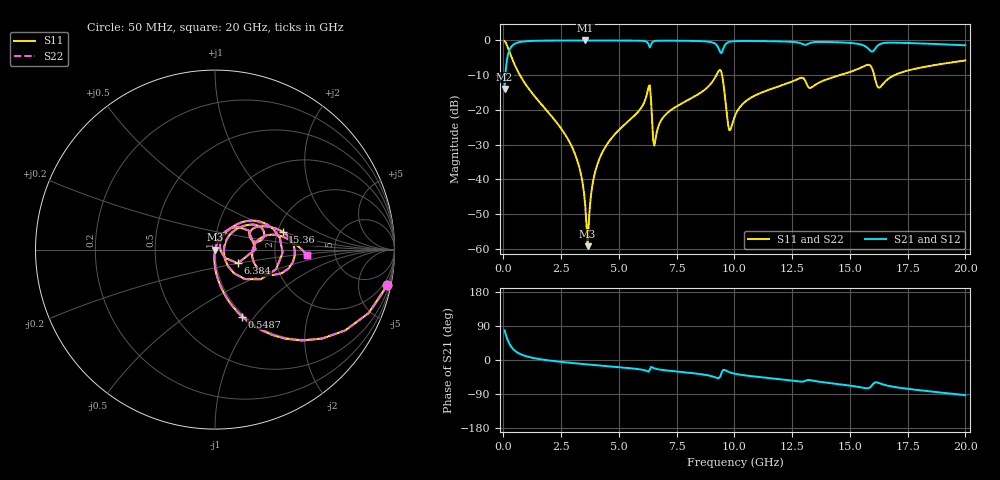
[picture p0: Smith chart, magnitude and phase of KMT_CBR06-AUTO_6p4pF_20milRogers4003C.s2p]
! Data measured by Modelithics Inc. support@modelithics.com 813-866-6335
! KEMET CBR06-AUTO 6.4pF, Pad Width= 0.851mm, Pad Length= 0.64mm, Pad Gap= 0.62mm, 20mil Rogers 4003C substrate Data, January 2022
# hz S ma R 50
! 2 Port Network Data from SP1.SP block
! freq  magS11  angS11  magS21  angS21  magS12  angS12  magS22  angS22
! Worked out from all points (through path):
!   401 points, 50 MHz to 20 GHz, reference 50 ohm
!   highest |S21| = -0.01 dB at 3.541 GHz (marker M1); lowest = -14.0 dB at 50 MHz (marker M2)
!   group delay of S21, straight-line fit = 14.4 ps
!   lowest |S11| = -59.3 dB at 3.641 GHz (marker M3), VSWR 1.00, Z = 50.1 - j0.0271 ohm
!   |S11| at or under -10 dB: 712.4 MHz to 9.218 GHz (8.505 GHz wide, 171 % of centre); 9.464 GHz to 14.57 GHz (5.107 GHz wide, 42.5 % of centre); 16.05 GHz to 16.93 GHz (880.3 MHz wide, 5.34 % of centre)
!   |S22| runs from -59.3 to -0.2 dB; largest |S21 - S12| = 0
!   S11 on the Smith chart (normalised r, x): 50 MHz: 0.98, -9.72; 548.8 MHz: 0.97, -0.87; 6.384 GHz: 1.27, -0.20; 15.36 GHz: 2.13, +0.50; 20 GHz: 3.09, -0.27
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5e7  0.98 -11.6  0.1989 78.4  0.1989 78.4  0.98 -11.6
2.495e8  0.7009 -46.3  0.7128 43.7  0.7128 43.7  0.7009 -46.3
5.4875e8  0.4021 -68.0  0.915 21.9  0.915 21.9  0.4021 -68.0
2.74325e9  0.04027 -95.1  0.9981 -6.5  0.9981 -6.5  0.04027 -95.1
3.391625e9  0.01028 -94.5  0.9988 -10.3  0.9988 -10.3  0.01028 -94.5
3.54125e9  0.004197 -86.4  0.9988 -11.1  0.9988 -11.1  0.004197 -86.4
3.641e9  0.001085 -14.4  0.9988 -11.7  0.9988 -11.7  0.001085 -14.4
3.94025e9  0.01162 71.1  0.9987 -13.3  0.9987 -13.3  0.01162 71.1
4.33925e9  0.0265 71.9  0.9983 -15.4  0.9983 -15.4  0.0265 71.9
6.2345e9  0.1807 44.3  0.9355 -29.9  0.9355 -29.9  0.1807 44.3
6.384125e9  0.1479 -31.1  0.8548 -18.5  0.8548 -18.5  0.1479 -31.1
6.53375e9  0.03052 21.4  0.9774 -22.0  0.9774 -22.0  0.03052 21.4
6.73325e9  0.0609 58.1  0.9905 -24.9  0.9905 -24.9  0.0609 58.1
9.32675e9  0.3673 10.0  0.7538 -47.7  0.7538 -47.7  0.3673 10.0
9.775625e9  0.05081 -11.4  0.9519 -32.0  0.9519 -32.0  0.05081 -11.4
1.0025e10  0.08199 39.5  0.9764 -36.3  0.9764 -36.3  0.08199 39.5
1.132175e10  0.1853 41.8  0.9767 -46.4  0.9767 -46.4  0.1853 41.8
1.336662e10  0.2129 25.1  0.9373 -54.1  0.9373 -54.1  0.2129 25.1
1.536162e10  0.3899 14.7  0.8912 -71.0  0.8912 -71.0  0.3899 14.7
1.601e10  0.3528 -23.7  0.7009 -62.9  0.7009 -62.9  0.3528 -23.7
1.670825e10  0.2874 15.4  0.9281 -68.7  0.9281 -68.7  0.2874 15.4
2e10  0.5143 -3.6  0.8499 -92.9  0.8499 -92.9  0.5143 -3.6
